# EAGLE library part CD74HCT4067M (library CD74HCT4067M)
Check prices
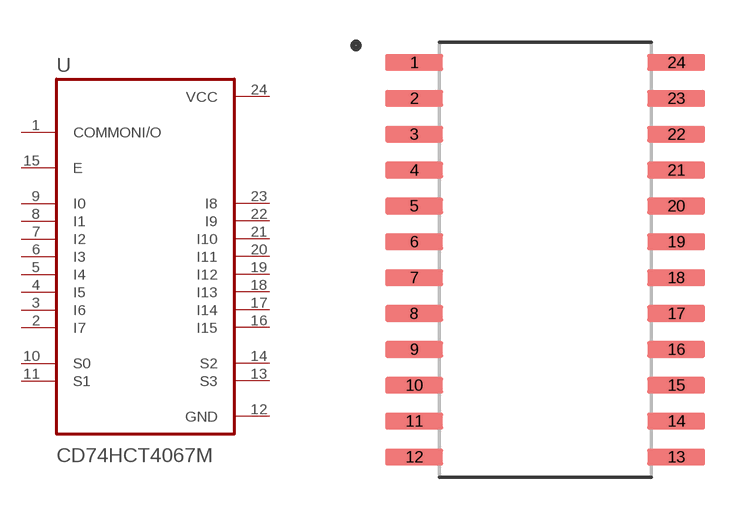
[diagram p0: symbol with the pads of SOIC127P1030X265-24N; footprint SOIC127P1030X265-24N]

Designator prefix U

## CD74HCT4067M (Availability: Good; Description: 5-V, 16:1, 1-channel analog multiplexer with TTL inputs 24-SOIC -55 to 125; MF: Texas Instruments; MP: CD74HCT4067M; Package: SOIC-24 Texas Instruments; Price: None; Purchase-URL: https://pricing.snapeda.com/search/part/CD74HCT4067M/?ref=eda)  [SOIC127P1030X265-24N]
1  COMMONI/O
2  I7
3  I6
4  I5
5  I4
6  I3
7  I2
8  I1
9  I0
10  S0
11  S1
12  GND  pwr
13  S3
14  S2
15  E
16  I15
17  I14
18  I13
19  I12
20  I11
21  I10
22  I9
23  I8
24  VCC  pwr

## Footprint SOIC127P1030X265-24N (pad centres in mm)
smd 2.06 x 0.6: 1 -4.64,6.985; 2 -4.64,5.715; 3 -4.64,4.445; 4 -4.64,3.175; 5 -4.64,1.905; 6 -4.64,0.635; 7 -4.64,-0.635; 8 -4.64,-1.905; 9 -4.64,-3.175; 10 -4.64,-4.445; 11 -4.64,-5.715; 12 -4.64,-6.985; 13 4.64,-6.985; 14 4.64,-5.715; 15 4.64,-4.445; 16 4.64,-3.175; 17 4.64,-1.905; 18 4.64,-0.635; 19 4.64,0.635; 20 4.64,1.905; 21 4.64,3.175; 22 4.64,4.445; 23 4.64,5.715; 24 4.64,6.985

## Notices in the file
This work is licensed under a Creative Commons Attribution-ShareAlike 4.0 International License (CC BY-SA) with Design Exception 1.0
